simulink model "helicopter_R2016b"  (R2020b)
settings: Solver=ode1  StartTime=0.0  StopTime=inf  FixedStep=0.002  RelTol=1e-3  EnableMultiTasking=on
PostLoadFcn:
  | qc_set_target_type(getConfigSet(bdroot, 'QUARC Default Target Configuration'));
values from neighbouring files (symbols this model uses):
  elevation_gain = 1    [init.m]
  K = dlqr(A1, B1, Q_lq, R_lq)    [template_problem_3.m]    (also in template_problem_4.m)
  K_ed = 2*d_e*sqrt(K_ep/K_3)    [init.m]
  K_ei = K_ep*0.1    (= 0.348080190282)    [init.m]
  K_ep = w_e^2/K_3    (= 3.48080190282)    [init.m]
  K_pd = 2*d_p*sqrt(K_pp/K_1)    [init.m]
  K_pp = w_p^2/K_1    (= 5.8991559633)    [init.m]
  travel_gain = 1    [init.m]
  Vd_ff = V_d_eq    (= 0.1)    [init.m]
  Vs_ff = V_s_eq    (= 7.88)    [init.m]
undefined symbols (not defined in the file or in its folder): HIL, qc_get_step_size
libraries: simulink_extras x9, quarc_library x3

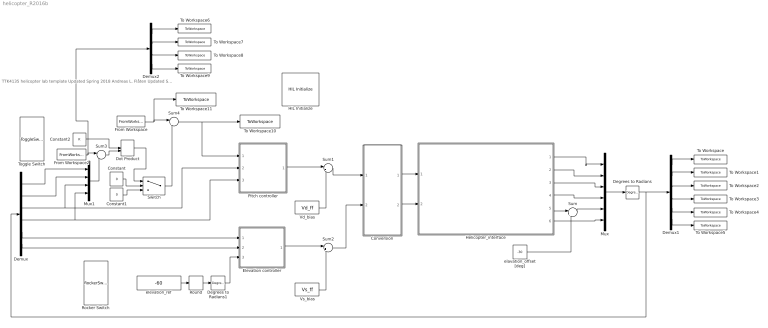
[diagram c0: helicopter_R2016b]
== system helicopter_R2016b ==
  note: TTK4135 helicopter lab template Updated Spring 2018 Andreas L. Flåten Updated Spring 2021 Joakim R. Andersen
  Constant : Constant  Value=0
  Constant1 : Constant  Value=0
  Constant2 : Constant  Value=K
  Conversion : Subsystem
  Degrees to Radians : simulink_extras/Transformations/Degrees to Radians
  Degrees to Radians1 : simulink_extras/Transformations/Degrees to Radians
  Demux : Demux  Outputs=6
  Demux1 : Demux  Outputs=6
  Demux2 : Demux
  Dot Product : DotProduct
  Elevation controller : Subsystem
  From Workspace : FromWorkspace  VariableName=u_opt_time
  From Workspace2 : FromWorkspace  VariableName=x_opt_time
  HIL Initialize : quarc_library/Data Acquisition/Generic/Configuration/HIL Initialize  Priority=-99  object_name=HIL-1  board_type=q8_usb  board_number=0  board_options=update_rate=normal;decimation=1  exclusive=off  active=off  hardware_clocks=[0:2]  clock_modes=[]  initial_clock_frequencies=[]  set_clock_params_at_start=off  set_clock_params_at_switch_in=off  set_clock_frequencies_at_start=off  set_clock_frequencies_at_switch_in=off  analog_input_channels=[0:7]  analog_input_configurations=[]  analog_input_maximums=10  analog_input_minimums=-10  set_analog_input_params_at_start=on  set_analog_input_params_at_switch_in=off  analog_output_channels=[0:7]  analog_output_maximums=10  analog_output_minimums=-10  initial_analog_outputs=[0]  final_analog_outputs=[0]  watchdog_analog_outputs=0  set_analog_output_params_at_start=on  set_analog_output_params_at_switch_in=off  set_analog_outputs_at_start=on  set_analog_outputs_at_switch_in=off  set_analog_outputs_at_terminate=on  set_analog_outputs_at_switch_out=off  set_analog_outputs_on_watchdog=off  digital_input_channels=[]  digital_output_channels=[]  digital_output_configuration=[]  initial_digital_outputs=[1]  final_digital_outputs=[1]  watchdog_digital_outputs=[1]  set_digital_output_params_at_start=off  set_digital_output_params_at_switch_in=off  set_digital_outputs_at_start=on  set_digital_outputs_at_switch_in=off  set_digital_outputs_at_terminate=on  set_digital_outputs_at_switch_out=off  set_digital_outputs_on_watchdog=off  encoder_channels=[0:7]  quadrature=[4]  encoder_filter_frequency=[]  initial_encoder_counts=[0]  set_encoder_params_at_start=on  set_encoder_params_at_switch_in=off  set_encoder_counts_at_start=on  set_encoder_counts_at_switch_in=off  pwm_channels=[0:7]  pwm_modes=0  pwm_frequency=99.532799999999995e6/4095  pwm_configuration=[0]  pwm_alignment=[0]  pwm_polarity=[1]  pwm_leading_deadband=[0]  pwm_trailing_deadband=[0]  initial_pwm_outputs=[0]  final_pwm_outputs=[0]  watchdog_pwm_outputs=[0]  set_pwm_params_at_start=on  set_pwm_params_at_switch_in=off  set_pwm_outputs_at_start=on  set_pwm_outputs_at_switch_in=off  set_pwm_outputs_at_terminate=on  set_pwm_outputs_at_switch_out=off  set_pwm_outputs_on_watchdog=off  other_output_channels=[]  initial_other_outputs=[]  final_other_outputs=[]  watchdog_other_outputs=[]  set_other_outputs_at_start=off  set_other_outputs_at_switch_in=off  set_other_outputs_at_terminate=off  set_other_outputs_at_switch_out=off  set_other_outputs_on_watchdog=off
  Helicopter_interface : Subsystem
  Mux : Mux  Inputs=6
  Mux1 : Mux
  Pitch controller : Subsystem
  Rocker Switch : RockerSwitchBlock
  Round : Rounding  Operator=round
  Sum : Sum  Inputs=|++
  Sum1 : Sum  Inputs=|++
  Sum2 : Sum  Inputs=|++
  Sum3 : Sum  Inputs=|-+
  Sum4 : Sum  Inputs=|+-
  Switch : Switch  Criteria=u2 > Threshold
  To Workspace : ToWorkspace  VariableName=sim_travel  SampleTime=-1
  To Workspace1 : ToWorkspace  VariableName=sim_travel_dot  SampleTime=-1
  To Workspace10 : ToWorkspace  VariableName=sim_u  SampleTime=-1
  To Workspace11 : ToWorkspace  VariableName=sim_u_ref  SampleTime=-1
  To Workspace2 : ToWorkspace  VariableName=sim_pitch  SampleTime=-1
  To Workspace3 : ToWorkspace  VariableName=sim_pitch_dot  SampleTime=-1
  To Workspace4 : ToWorkspace  VariableName=sim_elevation  SampleTime=-1
  To Workspace5 : ToWorkspace  VariableName=sim_elevation_dot  SampleTime=-1
  To Workspace6 : ToWorkspace  VariableName=sim_travel_ref  SampleTime=-1
  To Workspace7 : ToWorkspace  VariableName=sim_travel_dot_ref  SampleTime=-1
  To Workspace8 : ToWorkspace  VariableName=sim_pitch_ref  SampleTime=-1
  To Workspace9 : ToWorkspace  VariableName=sim_pitch_dot_ref  SampleTime=-1
  Toggle Switch : ToggleSwitchBlock
  Vd_bias : Constant  Value=Vd_ff
  Vs_bias : Constant  Value=Vs_ff
  elavation_offset [deg] : Constant  Value=-30
  elevation_ref : Constant  Value=-60
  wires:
  Conversion/2(Vb [V]) -> Helicopter_interface/2(Vb [V])
  Conversion/1(Vf [V]) -> Helicopter_interface/1(Vf [V])
  elavation_offset [deg]/1 -> Sum/2
  Helicopter_interface/5(Elevation [deg]) -> Sum/1
  Helicopter_interface/4(Pitch rate [deg/s]) -> Mux/4
  Helicopter_interface/3(Pitch [deg]) -> Mux/3
  Helicopter_interface/2(Travel rate [deg/s]) -> Mux/2
  Helicopter_interface/1(Travel [deg]) -> Mux/1
  Sum/1 -> Mux/5
  Helicopter_interface/6(Elevation rate [deg/s]) -> Mux/6
  Mux/1 -> Degrees to Radians/1
  Degrees to Radians/1 -> Demux/1, Demux1/1
  Demux/1 -> Mux1/1
  Demux/3 -> Pitch controller/2(p [rad]), Mux1/3
  Demux/4 -> Mux1/4, Pitch controller/3(p_dot [rad/s])
  Demux/6 -> Elevation controller/2(e_dot [rad/s])
  Demux/5 -> Elevation controller/1(e [rad])
  Vd_bias/1 -> Sum1/2
  Pitch controller/1(Vd [V]) -> Sum1/1
  Sum1/1 -> Conversion/1(Vd [V])
  Vs_bias/1 -> Sum2/2
  Sum2/1 -> Conversion/2(Vs [V])
  Elevation controller/1(Vs [V]) -> Sum2/1
  Constant/1 -> Switch/2
  Demux/2 -> Mux1/2
  Constant2/1 -> Dot Product/1
  From Workspace2/1 -> Demux2/1, Sum3/1
  Mux1/1 -> Sum3/2
  Sum3/1 -> Dot Product/2
  From Workspace/1 -> To Workspace11/1, Sum4/1
  Sum4/1 -> To Workspace10/1, Pitch controller/1(p_ref [rad])
  Dot Product/1 -> Switch/1
  Switch/1 -> Sum4/2
  Constant1/1 -> Switch/3
  Demux1/1 -> To Workspace/1
  Demux1/2 -> To Workspace1/1
  Demux1/3 -> To Workspace2/1
  Demux1/4 -> To Workspace3/1
  Demux1/5 -> To Workspace4/1
  Demux1/6 -> To Workspace5/1
  Round/1 -> Degrees to Radians1/1
  elevation_ref/1 -> Round/1
  Degrees to Radians1/1 -> Elevation controller/3(e_ref [rad])
  Demux2/4 -> To Workspace9/1
  Demux2/2 -> To Workspace7/1
  Demux2/1 -> To Workspace6/1
  Demux2/3 -> To Workspace8/1

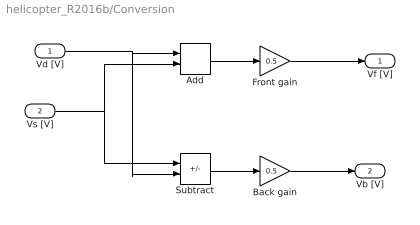
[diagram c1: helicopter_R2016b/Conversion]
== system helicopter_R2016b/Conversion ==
  Vd [V] : Inport
  Vs [V] : Inport  Port=2
  Add : Sum
  Back gain : Gain  Gain=0.5
  Front gain : Gain  Gain=0.5
  Subtract : Sum  Inputs=+-
  Vf [V] : Outport
  Vb [V] : Outport  Port=2
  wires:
  Vd [V]/1 -> Subtract/2, Add/1
  Vs [V]/1 -> Subtract/1, Add/2
  Subtract/1 -> Back gain/1
  Back gain/1 -> Vb [V]/1
  Add/1 -> Front gain/1
  Front gain/1 -> Vf [V]/1

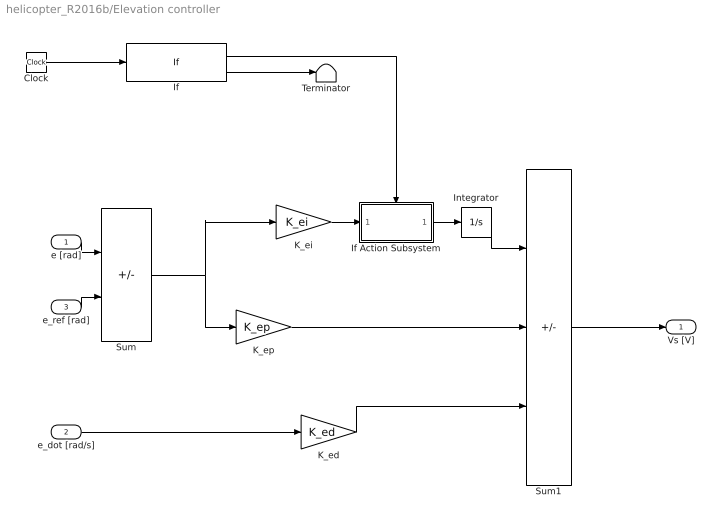
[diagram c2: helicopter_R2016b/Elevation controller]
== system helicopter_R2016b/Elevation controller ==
  e [rad] : Inport
  e_dot [rad/s] : Inport  Port=2
  e_ref [rad] : Inport  Port=3
  Clock : Clock
  If : If  IfExpression=u1 >=2
  If Action Subsystem : Subsystem  TreatAsAtomicUnit=on
  Integrator : Integrator  LimitOutput=on
  K_ed : Gain  Gain=K_ed  SaturateOnIntegerOverflow=on
  K_ei : Gain  Gain=K_ei  SaturateOnIntegerOverflow=on
  K_ep : Gain  Gain=K_ep  SaturateOnIntegerOverflow=on
  Sum : Sum  Inputs=-+  InputSameDT=on  SaturateOnIntegerOverflow=on
  Sum1 : Sum  Inputs=++-  InputSameDT=on  SaturateOnIntegerOverflow=on
  Terminator : Terminator
  Vs [V] : Outport  InitialOutput=0
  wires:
  K_ed/1 -> Sum1/3
  e_dot [rad/s]/1 -> K_ed/1
  Sum1/1 -> Vs [V]/1
  K_ei/1 -> If Action Subsystem/1(In1)
  If Action Subsystem/1(Out1) -> Integrator/1
  If/2 -> Terminator/1
  Clock/1 -> If/1
  e [rad]/1 -> Sum/1
  K_ep/1 -> Sum1/2
  e_ref [rad]/1 -> Sum/2
  Sum/1 -> K_ep/1, K_ei/1
  If/1 -> If Action Subsystem/Action
  Integrator/1 -> Sum1/1

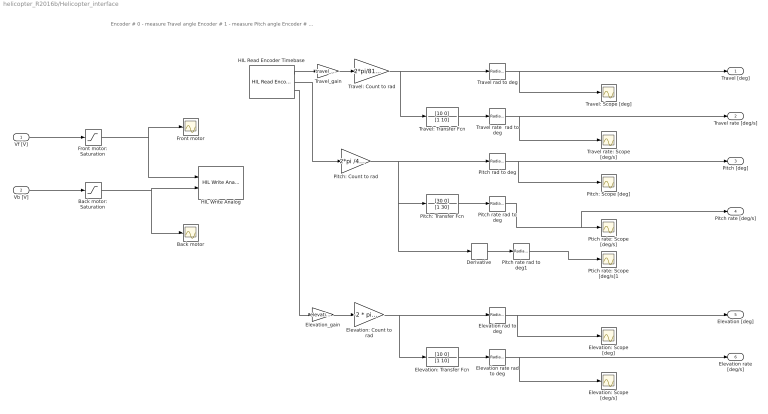
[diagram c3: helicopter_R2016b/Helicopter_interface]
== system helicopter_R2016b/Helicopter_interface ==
  note: Encoder # 0 - measure Travel angle Encoder # 1 - measure Pitch angle Encoder # 2 - measure Elavation angle
  Vf [V] : Inport
  Vb [V] : Inport  Port=2
  Back motor : Scope
  Back motor: Saturation : Saturate  UpperLimit=5  LowerLimit=-5
  Derivative : Derivative
  Elevation rad to deg : simulink_extras/Transformations/Radians to Degrees
  Elevation rate rad to deg : simulink_extras/Transformations/Radians to Degrees
  Elevation: Count to rad : Gain  Gain=-2 * pi /4096
  Elevation: Scope [deg/s] : Scope
  Elevation: Scope [deg] : Scope
  Elevation: Transfer Fcn : TransferFcn  Numerator=[10 0]  Denominator=[1 10]
  Elevation_gain : Gain  Gain=elevation_gain
  Front motor : Scope
  Front motor: Saturation : Saturate  UpperLimit=5  LowerLimit=-5
  HIL Read Encoder Timebase : quarc_library/Data Acquisition/Generic/Timebases/HIL Read Encoder Timebase  object_name=HIL-1  clock=0  channels=[0:2]  active=on  vector_output=off  data_type_mode=Inherit via back propagation  data_type=double  overflow_mode=Error on overflow  samples_in_buffer=max(ceil(1/qc_get_step_size), 1)
  HIL Write Analog : quarc_library/Data Acquisition/Generic/Immediate I//O/HIL Write Analog  object_name=HIL-1  channels=[0:1]  sample_time=-1  active=off  vector_input=off
  Pitch rad to deg : simulink_extras/Transformations/Radians to Degrees
  Pitch rate rad to deg : simulink_extras/Transformations/Radians to Degrees
  Pitch rate rad to deg1 : simulink_extras/Transformations/Radians to Degrees
  Pitch: Count to rad : Gain  Gain=2*pi /4096
  Pitch: Scope [deg] : Scope
  Pitch: Transfer Fcn : TransferFcn  Numerator=[30 0]  Denominator=[1 30]
  Ptich rate: Scope [deg/s] : Scope
  Ptich rate: Scope [deg/s]1 : Scope
  Travel rad to deg : simulink_extras/Transformations/Radians to Degrees
  Travel rate  rad to deg : simulink_extras/Transformations/Radians to Degrees
  Travel rate: Scope [deg/s] : Scope
  Travel: Count to rad : Gain  Gain=2*pi/8192
  Travel: Scope [deg] : Scope
  Travel: Transfer Fcn : TransferFcn  Numerator=[10 0]  Denominator=[1 10]
  Travel_gain : Gain  Gain=travel_gain
  Travel [deg] : Outport
  Travel rate [deg/s] : Outport  Port=2
  Pitch [deg] : Outport  Port=3
  Pitch rate [deg/s] : Outport  Port=4
  Elevation [deg] : Outport  Port=5
  Elevation rate [deg/s] : Outport  Port=6
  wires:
  HIL Read Encoder Timebase/1 -> Travel_gain/1
  HIL Read Encoder Timebase/2 -> Pitch: Count to rad/1
  HIL Read Encoder Timebase/3 -> Elevation_gain/1
  Travel: Count to rad/1 -> Travel: Transfer Fcn/1, Travel rad to deg/1
  Travel: Transfer Fcn/1 -> Travel rate  rad to deg/1
  Pitch: Transfer Fcn/1 -> Pitch rate rad to deg/1
  Elevation: Count to rad/1 -> Elevation: Transfer Fcn/1, Elevation rad to deg/1
  Elevation: Transfer Fcn/1 -> Elevation rate rad to deg/1
  Travel rad to deg/1 -> Travel: Scope [deg]/1, Travel [deg]/1
  Travel rate  rad to deg/1 -> Travel rate: Scope [deg/s]/1, Travel rate [deg/s]/1
  Vf [V]/1 -> Front motor: Saturation/1
  Vb [V]/1 -> Back motor: Saturation/1
  Front motor: Saturation/1 -> HIL Write Analog/1, Front motor/1
  Back motor: Saturation/1 -> Back motor/1, HIL Write Analog/2
  Derivative/1 -> Pitch rate rad to deg1/1
  Pitch: Count to rad/1 -> Derivative/1, Pitch: Transfer Fcn/1, Pitch rad to deg/1
  Pitch rate rad to deg1/1 -> Ptich rate: Scope [deg/s]1/1
  Pitch rad to deg/1 -> Pitch [deg]/1, Pitch: Scope [deg]/1
  Pitch rate rad to deg/1 -> Pitch rate [deg/s]/1, Ptich rate: Scope [deg/s]/1
  Elevation rad to deg/1 -> Elevation [deg]/1, Elevation: Scope [deg]/1
  Elevation rate rad to deg/1 -> Elevation rate [deg/s]/1, Elevation: Scope [deg/s]/1
  Travel_gain/1 -> Travel: Count to rad/1
  Elevation_gain/1 -> Elevation: Count to rad/1

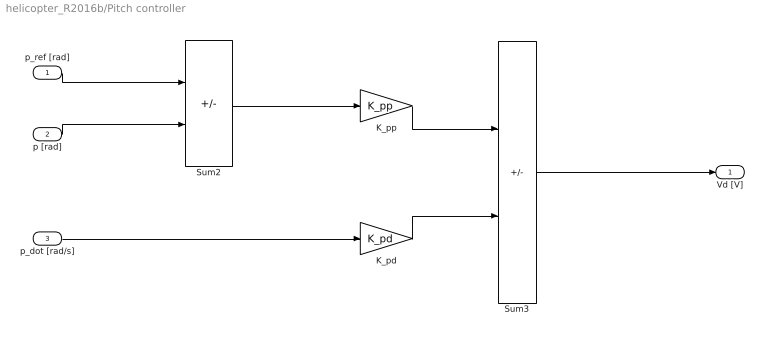
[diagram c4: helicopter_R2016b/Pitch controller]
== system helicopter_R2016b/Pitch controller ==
  p_ref [rad] : Inport
  p [rad] : Inport  Port=2
  p_dot [rad/s] : Inport  Port=3
  K_pd : Gain  Gain=K_pd  SaturateOnIntegerOverflow=on
  K_pp : Gain  Gain=K_pp  SaturateOnIntegerOverflow=on
  Sum2 : Sum  Inputs=+-  InputSameDT=on  SaturateOnIntegerOverflow=on
  Sum3 : Sum  Inputs=+-  InputSameDT=on  SaturateOnIntegerOverflow=on
  Vd [V] : Outport  InitialOutput=0
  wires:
  p_ref [rad]/1 -> Sum2/1
  p [rad]/1 -> Sum2/2
  p_dot [rad/s]/1 -> K_pd/1
  K_pp/1 -> Sum3/1
  Sum2/1 -> K_pp/1
  K_pd/1 -> Sum3/2
  Sum3/1 -> Vd [V]/1

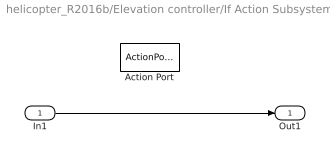
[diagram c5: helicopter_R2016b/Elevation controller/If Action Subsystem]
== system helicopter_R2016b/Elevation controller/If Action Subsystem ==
  In1 : Inport
  Action Port : ActionPort  ActionPortLabel=if(u1 >=2)
  Out1 : Outport
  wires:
  In1/1 -> Out1/1
